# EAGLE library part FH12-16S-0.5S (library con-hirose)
0.5mm Pitch Connectors For FPC/FFC Source: Data sheet
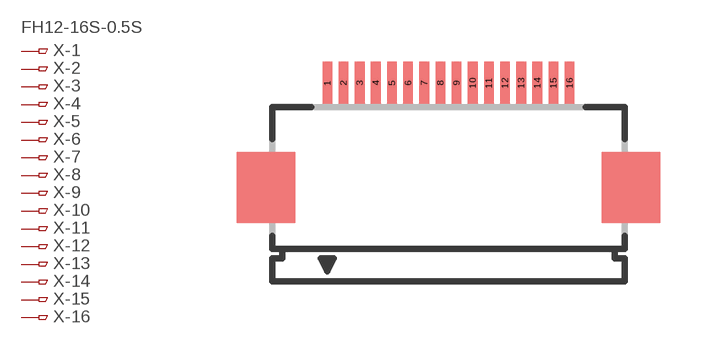
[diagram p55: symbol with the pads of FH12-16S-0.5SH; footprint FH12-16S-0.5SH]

Designator prefix X; gates -1=PINV -2=PIN -3=PIN -4=PIN -5=PIN -6=PIN -7=PIN -8=PIN -9=PIN -10=PIN -11=PIN -12=PIN -13=PIN -14=PIN -15=PIN -16=PIN

## FH12-16S-0.5SH (MPN: FH12-16S-0.5SH(55); OC_FARNELL: 1324546; OC_NEWARK: 34M6162)  [FH12-16S-0.5SH]
1  -1:1  pas
2  -2:1  pas
3  -3:1  pas
4  -4:1  pas
5  -5:1  pas
6  -6:1  pas
7  -7:1  pas
8  -8:1  pas
9  -9:1  pas
10  -10:1  pas
11  -11:1  pas
12  -12:1  pas
13  -13:1  pas
14  -14:1  pas
15  -15:1  pas
16  -16:1  pas

## Footprint FH12-16S-0.5SH (pad centres in mm)
0.5mm Pitch Connectors For FPC/FFC Source: Data sheet
smd 0.3 x 1.3: 1 -3.75,3.25; 2 -3.25,3.25; 3 -2.75,3.25; 4 -2.25,3.25; 5 -1.75,3.25; 6 -1.25,3.25; 7 -0.75,3.25; 8 -0.25,3.25; 9 0.25,3.25; 10 0.75,3.25; 11 1.25,3.25; 12 1.75,3.25; 13 2.25,3.25; 14 2.75,3.25; 15 3.25,3.25; 16 3.75,3.25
